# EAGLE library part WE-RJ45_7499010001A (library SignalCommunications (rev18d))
Order Code 7499010001A Design THT xBase-T 10/100 Base-T Ports 1x1 Application Standard Tab Position UP LED (Left-Right) NONE EMI Fingers No Details see: http://katalog.we-online.de/en/pbs/WE-LAN_RJ45/7499010001A? Updated by Yingchun Shan 2016-08-26 2016(C) Würth Elektronik
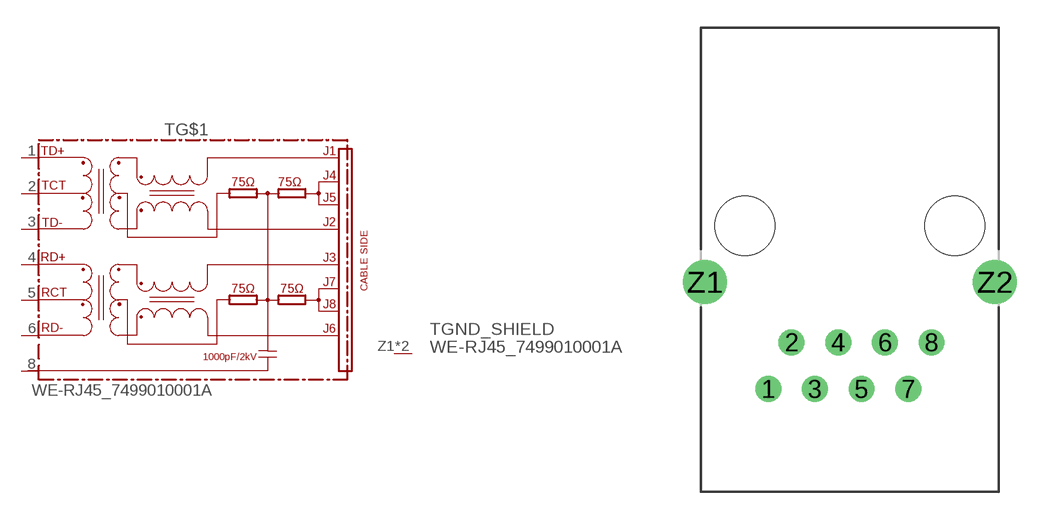
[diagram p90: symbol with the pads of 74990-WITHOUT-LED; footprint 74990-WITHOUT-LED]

Designator prefix T; gates GND_SHIELD=GNDPIN G$1=74990X-THT-10/100-T

## WE-RJ45_7499010001A (COMPANY-URL: http://www.we-online.de; CREATED-BY: Christin Zierenner; CREATED-DATE: AUG 2012; DATASHEET-URL: http://katalog.we-online.de/kataloge/eisos/media/pdf/7499010001A.pdf; MANUFACTURER: Würth Elektronik eiSos GmbH)  [74990-WITHOUT-LED]
1  G$1:TD+
2  G$1:TCT
3  G$1:TD-
4  G$1:RD+
5  G$1:RCT
6  G$1:RD-
8  G$1:8
Z1  GND_SHIELD:GND  pwr
Z2  GND_SHIELD:GND  pwr

## Footprint 74990-WITHOUT-LED (pad centres in mm)
MAX HEIGHT=13.50mm PORTS----1X1 LED ----NO
drill 0.9: 1 -4.445,-8.89; 2 -3.175,-6.35; 3 -1.905,-8.89; 4 -0.635,-6.35; 5 0.635,-8.89; 6 1.905,-6.35; 7 3.175,-8.89; 8 4.445,-6.35
drill 1.6: Z1 -7.9,-3.05; Z2 7.9,-3.05
hole 3.25 at 5.715,0
hole 3.25 at -5.715,0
